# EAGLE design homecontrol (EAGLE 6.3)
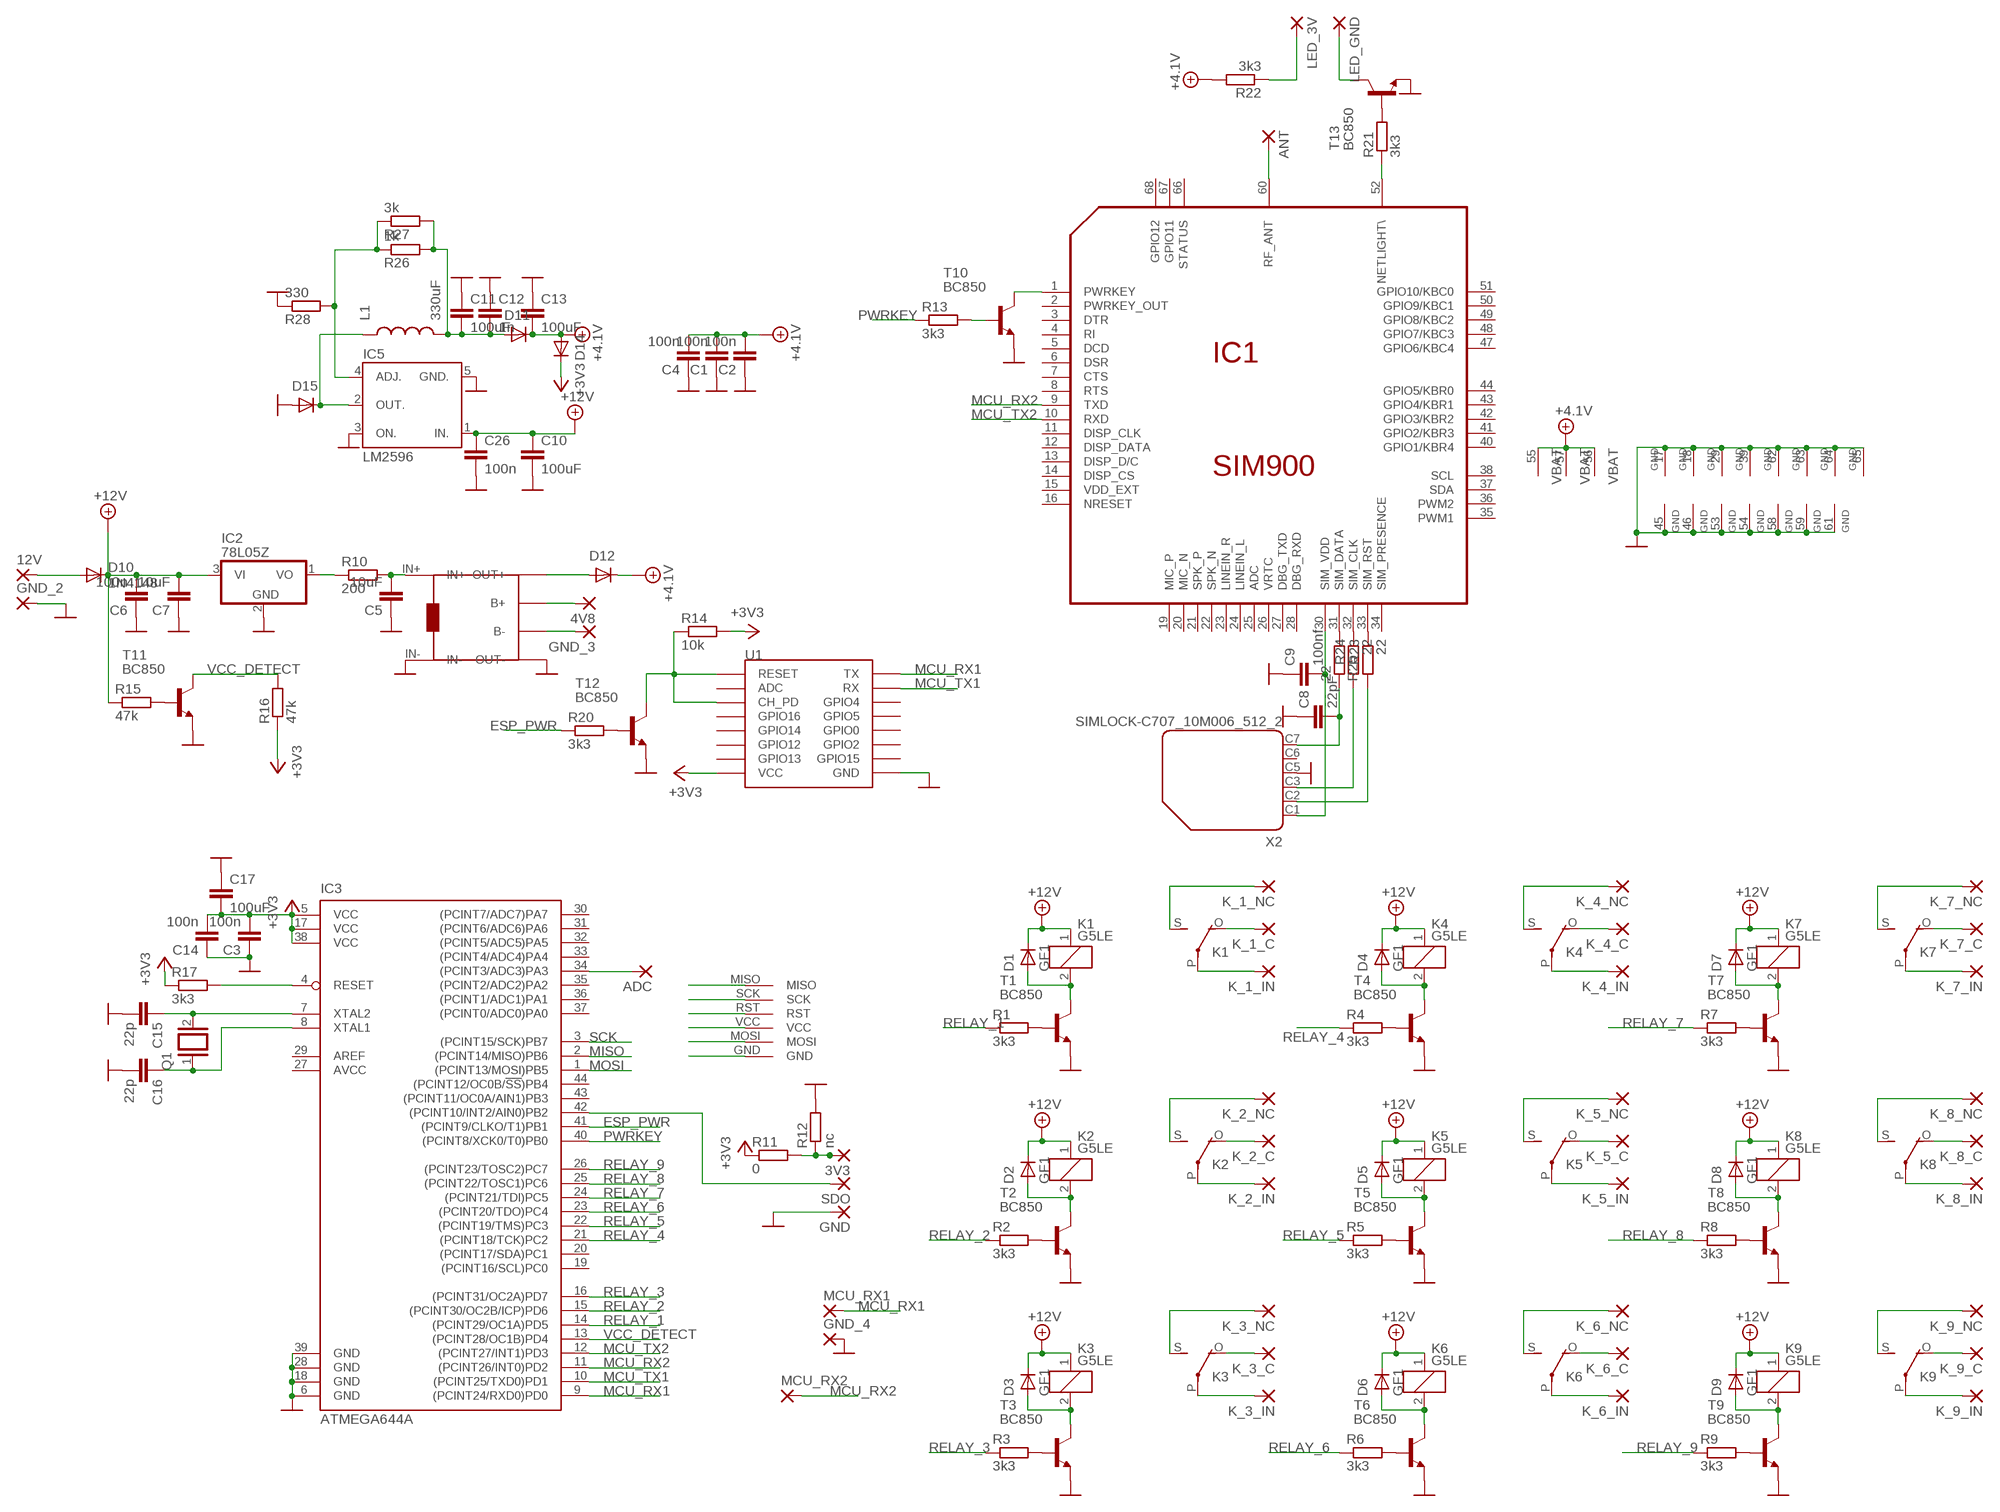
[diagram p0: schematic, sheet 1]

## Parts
3V3  2,15/1,0  [2,15/1,0]
4V8  WIREPAD2,15/1,0  [2,15/1,0]
12V  2,54/0,8  [2,54/0,8]
ADC  SMD2  [SMD1,27-2,54]
ANT  2,54/0,8  [2,54/0,8]
C1  100n  C-EUC1206  [C1206]
C2  100n  C-EUC1206  [C1206]
C3  100n  C-EUC1206  [C1206]
C4  100n  C-EUC1206  [C1206]
C5  10uF  C-EUC1206  [C1206]
C6  100n  C-EUC1206  [C1206]
C7  10uF  C-EUC1206  [C1206]
C8  22pF  C-EUC1206K  [C1206K]
C9  100nf  C-EUC1206K  [C1206K]
C10  100uF  SMD-CAP  [SMD-CAP]
C11  100uF  SMD-CAP  [SMD-CAP]
C12  1n  C-EUC1206K  [C1206K]
C13  100uF  SMD-CAP  [SMD-CAP]
C14  100n  C-EUC1206  [C1206]
C15  22p  C-EUC1206  [C1206]
C16  22p  C-EUC1206  [C1206]
C17  100uF  SMD-CAP  [SMD-CAP]
C26  100n  C-EUC1206K  [C1206K]
D1  GF1  [SMA-DO214AC]
D2  GF1  [SMA-DO214AC]
D3  GF1  [SMA-DO214AC]
D4  GF1  [SMA-DO214AC]
D5  GF1  [SMA-DO214AC]
D6  GF1  [SMA-DO214AC]
D7  GF1  [SMA-DO214AC]
D8  GF1  [SMA-DO214AC]
D9  GF1  [SMA-DO214AC]
D10  1N4148  1N4148DO35-10  [DO35-10]
D11  GF1  [SMA-DO214AC]
D12  GF1  [SMA-DO214AC]
D14  GF1  [SMA-DO214AC]
D15  GF1  [SMA-DO214AC]
GND  2,54/0,8  [2,54/0,8]
GND_2  2,15/1,0  [2,15/1,0]
GND_3  2,15/1,0  [2,15/1,0]
GND_4  2,15/1,0  [2,15/1,0]
IC1  SIM900  [SIM900]
IC2  78L05Z  [TO92]
IC3  ATMEGA644A  [TQFP44]
IC5  LM2596  LM2931S-ADJ  [TO263-5]
K1  G5LE  [G5LE]
K2  G5LE  [G5LE]
K3  G5LE  [G5LE]
K4  G5LE  [G5LE]
K5  G5LE  [G5LE]
K6  G5LE  [G5LE]
K7  G5LE  [G5LE]
K8  G5LE  [G5LE]
K9  G5LE  [G5LE]
K_1_C  2,54/0,8  [2,54/0,8]
K_1_IN  2,54/0,8  [2,54/0,8]
K_1_NC  2,54/0,8  [2,54/0,8]
K_2_C  2,54/0,8  [2,54/0,8]
K_2_IN  2,54/0,8  [2,54/0,8]
K_2_NC  2,54/0,8  [2,54/0,8]
K_3_C  2,54/0,8  [2,54/0,8]
K_3_IN  2,54/0,8  [2,54/0,8]
K_3_NC  2,54/0,8  [2,54/0,8]
K_4_C  2,54/0,8  [2,54/0,8]
K_4_IN  2,54/0,8  [2,54/0,8]
K_4_NC  2,54/0,8  [2,54/0,8]
K_5_C  2,54/0,8  [2,54/0,8]
K_5_IN  2,54/0,8  [2,54/0,8]
K_5_NC  2,54/0,8  [2,54/0,8]
K_6_C  2,54/0,8  [2,54/0,8]
K_6_IN  2,54/0,8  [2,54/0,8]
K_6_NC  2,54/0,8  [2,54/0,8]
K_7_C  2,54/0,8  [2,54/0,8]
K_7_IN  2,54/0,8  [2,54/0,8]
K_7_NC  2,54/0,8  [2,54/0,8]
K_8_C  2,54/0,8  [2,54/0,8]
K_8_IN  2,54/0,8  [2,54/0,8]
K_8_NC  2,54/0,8  [2,54/0,8]
K_9_C  2,54/0,8  [2,54/0,8]
K_9_IN  2,54/0,8  [2,54/0,8]
K_9_NC  2,54/0,8  [2,54/0,8]
L1  330uF  SMD-INDUCTOR  [SMD-COIL]
LED_3V  WIREPAD2,15/1,0  [2,15/1,0]
LED_GND  WIREPAD2,15/1,0  [2,15/1,0]
MCU_RX1  2,15/1,0  [2,15/1,0]
MCU_RX2  2,15/1,0  [2,15/1,0]
Q1  XTAL/S  [QS]
R1  3k3  R-EU_M3216  [M3216]
R2  3k3  R-EU_M3216  [M3216]
R3  3k3  R-EU_M3216  [M3216]
R4  3k3  R-EU_M3216  [M3216]
R5  3k3  R-EU_M3216  [M3216]
R6  3k3  R-EU_M3216  [M3216]
R7  3k3  R-EU_M3216  [M3216]
R8  3k3  R-EU_M3216  [M3216]
R9  3k3  R-EU_M3216  [M3216]
R10  200  R-EU_M3216  [M3216]
R11  0  R-EU_M3216  [M3216]
R12  nc  R-EU_M3216  [M3216]
R13  3k3  R-EU_M3216  [M3216]
R14  10k  R-EU_M3216  [M3216]
R15  47k  R-EU_M3216  [M3216]
R16  47k  R-EU_M3216  [M3216]
R17  3k3  R-EU_M3216  [M3216]
R20  3k3  R-EU_M3216  [M3216]
R21  3k3  R-EU_M3216  [M3216]
R22  3k3  R-EU_M3216  [M3216]
R23  22  R-EU_M1206  [M1206]
R24  22  R-EU_M1206  [M1206]
R25  22  R-EU_M1206  [M1206]
R26  1k  R-EU_M3216  [M3216]
R27  3k  R-EU_M3216  [M3216]
R28  330  R-EU_M3216  [M3216]
SDO  2,15/1,0  [2,15/1,0]
T1  BC850  [SOT23]
T2  BC850  [SOT23]
T3  BC850  [SOT23]
T4  BC850  [SOT23]
T5  BC850  [SOT23]
T6  BC850  [SOT23]
T7  BC850  [SOT23]
T8  BC850  [SOT23]
T9  BC850  [SOT23]
T10  BC850  [SOT23]
T11  BC850  [SOT23]
T12  BC850  [SOT23]
T13  BC850  [SOT23]
U1  ESP12SMD  [ESP12-SMD]
U$1  AVR_ISP  [AVR_ISP]
U$2  AKUTOLTO  [AKUTOLTO]
X2  SIMLOCK-C707_10M006_512_2  [C707_10M006_512_2]

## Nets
+3V3: C3.2 C14.2 C17.P$2 D14.K(C) IC3.5(VCC) IC3.17(VCC) IC3.38(VCC) R11.1 R14.2 R16.1 R17.1 U1.VCC U$1.VCC
+4.1V: C1.2 C2.2 C4.2 C13.P$2 D11.K(C) D12.K(C) D14.A IC1.55(VBAT) IC1.56(VBAT) IC1.57(VBAT) R22.2
+12V: C6.2 C7.2 C10.P$1 C26.1 D1.K(C) D2.K(C) D3.K(C) D4.K(C) D5.K(C) D6.K(C) D7.K(C) D8.K(C) D9.K(C) D10.C IC2.3(VI) IC5.1(IN.) K1.1 K2.1 K3.1 K4.1 K5.1 K6.1 K7.1 K8.1 K9.1 R15.1
ESP_PWR: IC3.41((PCINT9/CLKO/T1)PB1) R20.1
GND: C1.1 C2.1 C3.1 C4.1 C5.1 C6.1 C7.1 C8.1 C9.1 C10.P$2 C11.P$1 C12.1 C13.P$1 C14.1 C15.2 C16.2 C17.P$1 C26.2 D15.A GND.1(P) GND_2.1(P) GND_4.1(P) IC1.17(GND) IC1.18(GND) IC1.29(GND) IC1.39(GND) IC1.45(GND) IC1.46(GND) IC1.53(GND) IC1.54(GND) IC1.58(GND) IC1.59(GND) IC1.61(GND) IC1.62(GND) IC1.63(GND) IC1.64(GND) IC1.65(GND) IC2.2(GND) IC3.6(GND) IC3.18(GND) IC3.28(GND) IC3.39(GND) IC5.3(ON.) IC5.5(GND.) R12.2 R28.1 T1.2(E) T2.2(E) T3.2(E) T4.2(E) T5.2(E) T6.2(E) T7.2(E) T8.2(E) T9.2(E) T10.2(E) T11.2(E) T12.2(E) T13.2(E) U1.GND U$1.GND U$2.IN- U$2.OUT- X2.C5
MCU_RX1: IC3.9((PCINT24/RXD0)PD0) MCU_RX1.1(P) U1.TXD0(TX)
MCU_RX2: IC1.9(TXD) IC3.11((PCINT26/INT0)PD2) MCU_RX2.1(P)
MCU_TX1: IC3.10((PCINT25/TXD0)PD1) U1.RXD0(RX)
MCU_TX2: IC1.10(RXD) IC3.12((PCINT27/INT1)PD3)
MISO: IC3.2((PCINT14/MISO)PB6) U$1.MISO
MOSI: IC3.1((PCINT13/MOSI)PB5) U$1.MOSI
N$1: R1.2 T1.1(B)
N$2: D1.A K1.2 T1.3(C)
N$3: K1.S(2:S) K_1_NC.1(P)
N$4: K1.P(2:P) K_1_IN.1(P)
N$5: K1.O(2:O) K_1_C.1(P)
N$6: R2.2 T2.1(B)
N$7: D2.A K2.2 T2.3(C)
N$8: K2.P(2:P) K_2_IN.1(P)
N$9: K2.O(2:O) K_2_C.1(P)
N$10: K2.S(2:S) K_2_NC.1(P)
N$11: R3.2 T3.1(B)
N$12: D3.A K3.2 T3.3(C)
N$13: K3.P(2:P) K_3_IN.1(P)
N$14: K3.O(2:O) K_3_C.1(P)
N$15: K3.S(2:S) K_3_NC.1(P)
N$16: R4.2 T4.1(B)
N$17: D4.A K4.2 T4.3(C)
N$18: K4.P(2:P) K_4_IN.1(P)
N$19: K4.O(2:O) K_4_C.1(P)
N$20: K4.S(2:S) K_4_NC.1(P)
N$21: R5.2 T5.1(B)
N$22: D5.A K5.2 T5.3(C)
N$23: K5.P(2:P) K_5_IN.1(P)
N$24: K5.O(2:O) K_5_C.1(P)
N$25: K5.S(2:S) K_5_NC.1(P)
N$26: R6.2 T6.1(B)
N$27: D6.A K6.2 T6.3(C)
N$28: K6.P(2:P) K_6_IN.1(P)
N$29: K6.O(2:O) K_6_C.1(P)
N$30: K6.S(2:S) K_6_NC.1(P)
N$31: R7.2 T7.1(B)
N$32: D7.A K7.2 T7.3(C)
N$33: K7.P(2:P) K_7_IN.1(P)
N$34: K7.O(2:O) K_7_C.1(P)
N$35: K7.S(2:S) K_7_NC.1(P)
N$36: R8.2 T8.1(B)
N$37: D8.A K8.2 T8.3(C)
N$38: K8.P(2:P) K_8_IN.1(P)
N$39: K8.O(2:O) K_8_C.1(P)
N$40: K8.S(2:S) K_8_NC.1(P)
N$41: R9.2 T9.1(B)
N$42: D9.A K9.2 T9.3(C)
N$43: K9.P(2:P) K_9_IN.1(P)
N$44: K9.O(2:O) K_9_C.1(P)
N$45: K9.S(2:S) K_9_NC.1(P)
N$46: C5.2 R10.2 U$2.IN+
N$47: D12.A U$2.OUT+
N$48: IC2.1(VO) R10.1
N$49: IC3.42((PCINT10/INT2/AIN0)PB2) SDO.1(P)
N$50: 3V3.1(P) R11.2 R12.1
N$51: R13.2 T10.1(B)
N$52: IC1.1(PWRKEY) T10.3(C)
N$53: D15.K(C) IC5.2(OUT.) L1.P$1
N$54: 12V.1(P) D10.A
N$55: R14.1 T12.3(C) U1.CH_PD U1.RESET
N$56: 4V8.1(P) U$2.B+
N$57: R15.2 T11.1(B)
N$58: GND_3.1(P) U$2.B-
N$60: C11.P$2 C12.2 D11.A L1.P$2 R26.2 R27.2
N$61: C15.1 IC3.7(XTAL2) Q1.2
N$62: R20.2 T12.1(B)
N$63: IC5.4(ADJ.) R26.1 R27.1 R28.2
N$64: ANT.1(P) IC1.60(RF_ANT)
N$65: IC1.52(NETLIGHT\) R21.1
N$66: R21.2 T13.1(B)
N$67: LED_GND.1(P) T13.3(C)
N$68: LED_3V.1(P) R22.1
N$69: C9.2 IC1.30(SIM_VDD) X2.C1
N$70: R23.2 X2.C2
N$71: R24.2 X2.C3
N$72: C8.2 R25.1 X2.C7
N$73: IC1.33(SIM_RST) R23.1
N$74: IC1.32(SIM_CLK) R24.1
N$75: IC1.31(SIM_DATA) R25.2
N$79: C16.1 IC3.8(XTAL1) Q1.1
N$80: ADC.1(P) IC3.34((PCINT3/ADC3)PA3)
PWRKEY: IC3.40((PCINT8/XCK0/T0)PB0) R13.1
RELAY_1: IC3.14((PCINT29/OC1A)PD5) R1.1
RELAY_2: IC3.15((PCINT30/OC2B/ICP)PD6) R2.1
RELAY_3: IC3.16((PCINT31/OC2A)PD7) R3.1
RELAY_4: IC3.21((PCINT18/TCK)PC2) R4.1
RELAY_5: IC3.22((PCINT19/TMS)PC3) R5.1
RELAY_6: IC3.23((PCINT20/TDO)PC4) R6.1
RELAY_7: IC3.24((PCINT21/TDI)PC5) R7.1
RELAY_8: IC3.25((PCINT22/TOSC1)PC6) R8.1
RELAY_9: IC3.26((PCINT23/TOSC2)PC7) R9.1
RESET: IC3.4(RESET) R17.2 U$1.RST
SCK: IC3.3((PCINT15/SCK)PB7) U$1.SCK
VCC_DETECT: IC3.13((PCINT28/OC1B)PD4) R16.2 T11.3(C)
Unconnected: IC1.2(PWRKEY_OUT) IC1.3(DTR) IC1.4(RI) IC1.5(DCD) IC1.6(DSR) IC1.7(CTS) IC1.8(RTS) IC1.11(DISP_CLK) IC1.12(DISP_DATA) IC1.13(DISP_D/C) IC1.14(DISP_CS) IC1.15(VDD_EXT) IC1.16(NRESET) IC1.19(MIC_P) IC1.20(MIC_N) IC1.21(SPK_P) IC1.22(SPK_N) IC1.23(LINEIN_R) IC1.24(LINEIN_L) IC1.25(ADC) IC1.26(VRTC) IC1.27(DBG_TXD) IC1.28(DBG_RXD) IC1.34(SIM_PRESENCE) IC1.35(PWM1) IC1.36(PWM2) IC1.37(SDA) IC1.38(SCL) IC1.40(GPIO1/KBR4) IC1.41(GPIO2/KBR3) IC1.42(GPIO3/KBR2) IC1.43(GPIO4/KBR1) IC1.44(GPIO5/KBR0) IC1.47(GPIO6/KBC4) IC1.48(GPIO7/KBC3) IC1.49(GPIO8/KBC2) IC1.50(GPIO9/KBC1) IC1.51(GPIO10/KBC0) IC1.66(STATUS) IC1.67(GPIO11) IC1.68(GPIO12) IC3.19((PCINT16/SCL)PC0) IC3.20((PCINT17/SDA)PC1) IC3.29(AREF) IC3.30((PCINT7/ADC7)PA7) IC3.31((PCINT6/ADC6)PA6) IC3.32((PCINT5/ADC5)PA5) IC3.33((PCINT4/ADC4)PA4) IC3.35((PCINT2/ADC2)PA2) IC3.36((PCINT1/ADC1)PA1) IC3.37((PCINT0/ADC0)PA0) IC3.43((PCINT11/OC0A/AIN1)PB3) IC3.44((PCINT12/OC0B/!SS!)PB4) U1.ADC U1.GPIO0 U1.GPIO2 U1.GPIO4 U1.GPIO5 U1.GPIO12 U1.GPIO13 U1.GPIO14 U1.GPIO15 U1.GPIO16 X2.C6

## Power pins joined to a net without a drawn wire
AVCC: IC3.27(AVCC)

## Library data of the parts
3V3 GND_2-GND_4 MCU_RX1 MCU_RX2 SDO = wirepad:2,15/1,0: THROUGH-HOLE PAD
4V8 LED_3V LED_GND = wirepad:WIREPAD: Wire PAD connect wire on PCB
12V ANT GND K_1_C K_1_IN K_1_NC K_2_C K_2_IN K_2_NC K_3_C K_3_IN K_3_NC K_4_C K_4_IN K_4_NC K_5_C K_5_IN K_5_NC K_6_C K_6_IN K_6_NC K_7_C K_7_IN K_7_NC K_8_C K_8_IN K_8_NC K_9_C K_9_IN K_9_NC = wirepad:2,54/0,8: THROUGH-HOLE PAD
ADC = wirepad:SMD2: SMD PAD
C1-C7 C14-C16 = resistor:C-EU: CAPACITOR, European symbol
C8 C9 C12 C26 = rcl:C-EU: CAPACITOR, European symbol
C10 C11 C13 C17 = Tomi's_Library:SMD-CAP
D1-D9 D11 D12 D14 D15 = diode:GF1: DIODE
D10 = diode:1N4148: DIODE
IC1 = sim900:SIM900
IC2 = linear:78*: Positive VOLTAGE REGULATOR Source: http://cache.national.com/ds/LM/LM78L05.pdf http://www.fairchildsemi.com/ds/LM/LM7805.pdf
IC3 = atmel:ATMEGA644: 8-bit Microcontroller with 64K Bytes In-System Programmable Flash Source: http://www.atmel.com/dyn/resources/prod_documents/doc2593.pdf; MPN: ATMEGA644PV-10AU; OC_FARNELL: 1455123; OC_NEWARK: 58M3748
IC5 = regulator:LM2931?-ADJ: National Semiconductor Low Dropout Adjustable Regulator Vout 3-24V, Vin up to 26V, Shutdown Pin, Reverse Batterie/Load Dump/Short Circuit/Overload Protection,
K1-K9 = relay:G5LE: RELAY 1 x switch, 10 A/120 V AC, 8 A/30 V DC, Omron; OC_FARNELL: unknown; OC_NEWARK: unknown
L1 = Tomi's_Library:SMD-INDUCTOR
Q1 = special:XTAL/S: CRYSTAL
R1-R17 R20-R22 = rcl:R-EU_: RESISTOR, European symbol
R23-R28 = resistor:R-EU_: RESISTOR, European symbol
T1-T13 = transistor:BC850: NPN TRANSISTOR
U1 = esp8266modules:ESP12: ESP8266 Wifi module 12
U$1 = 2 - csatlakozo:AVR_ISP
U$2 = aksitolto:AKUTOLTO
X2 = con-amphenol:SIMLOCK-C707_10M006_512_2: C707A SIMLOCK® 2.5 mm with wide solder tails Source: Data sheet; OC_FARNELL: unknown; OC_NEWARK: unknown

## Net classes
0 default: clearance 0.355 mm

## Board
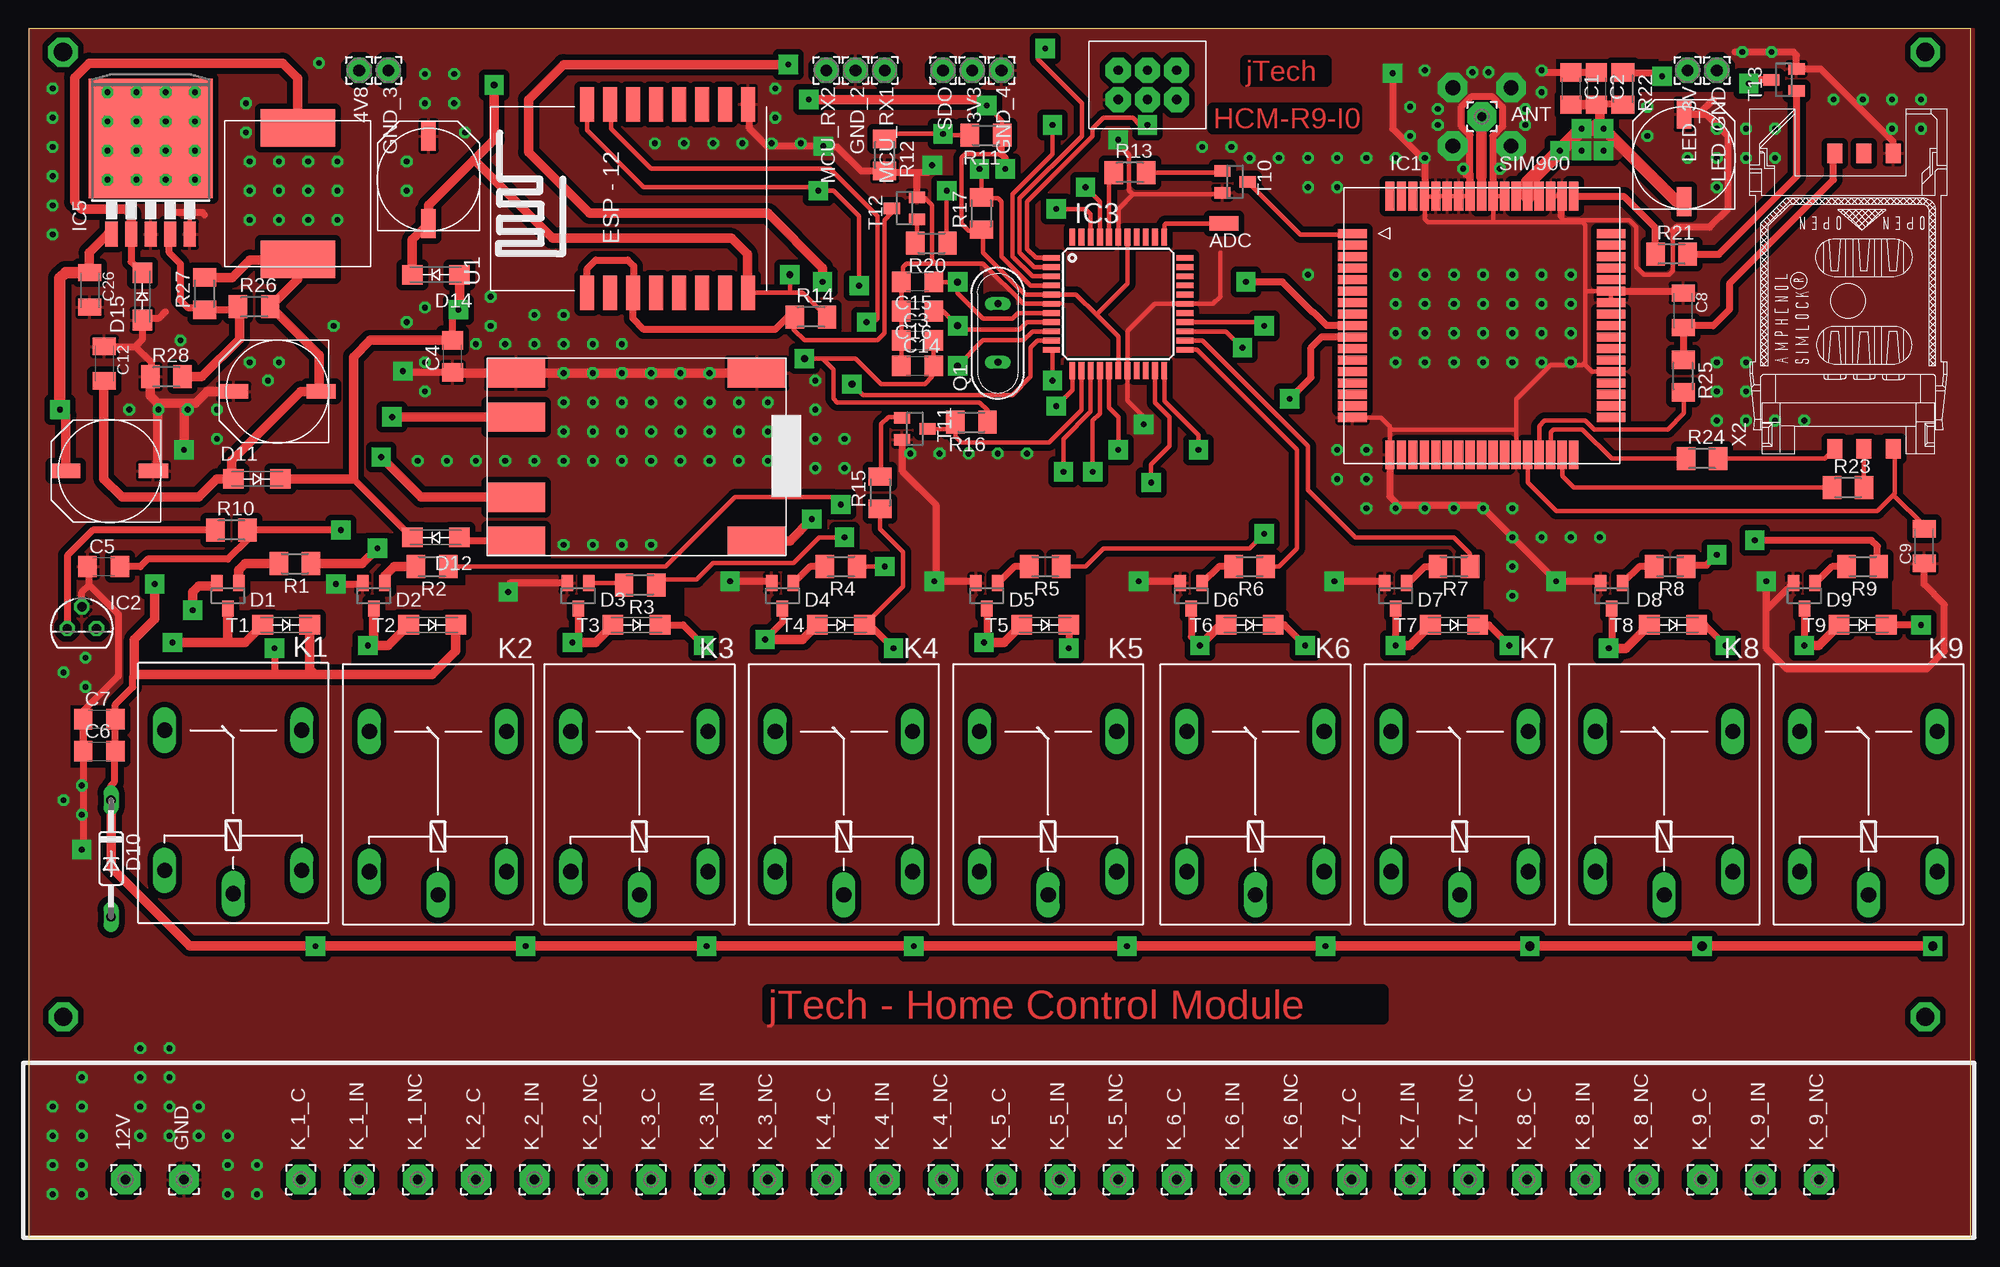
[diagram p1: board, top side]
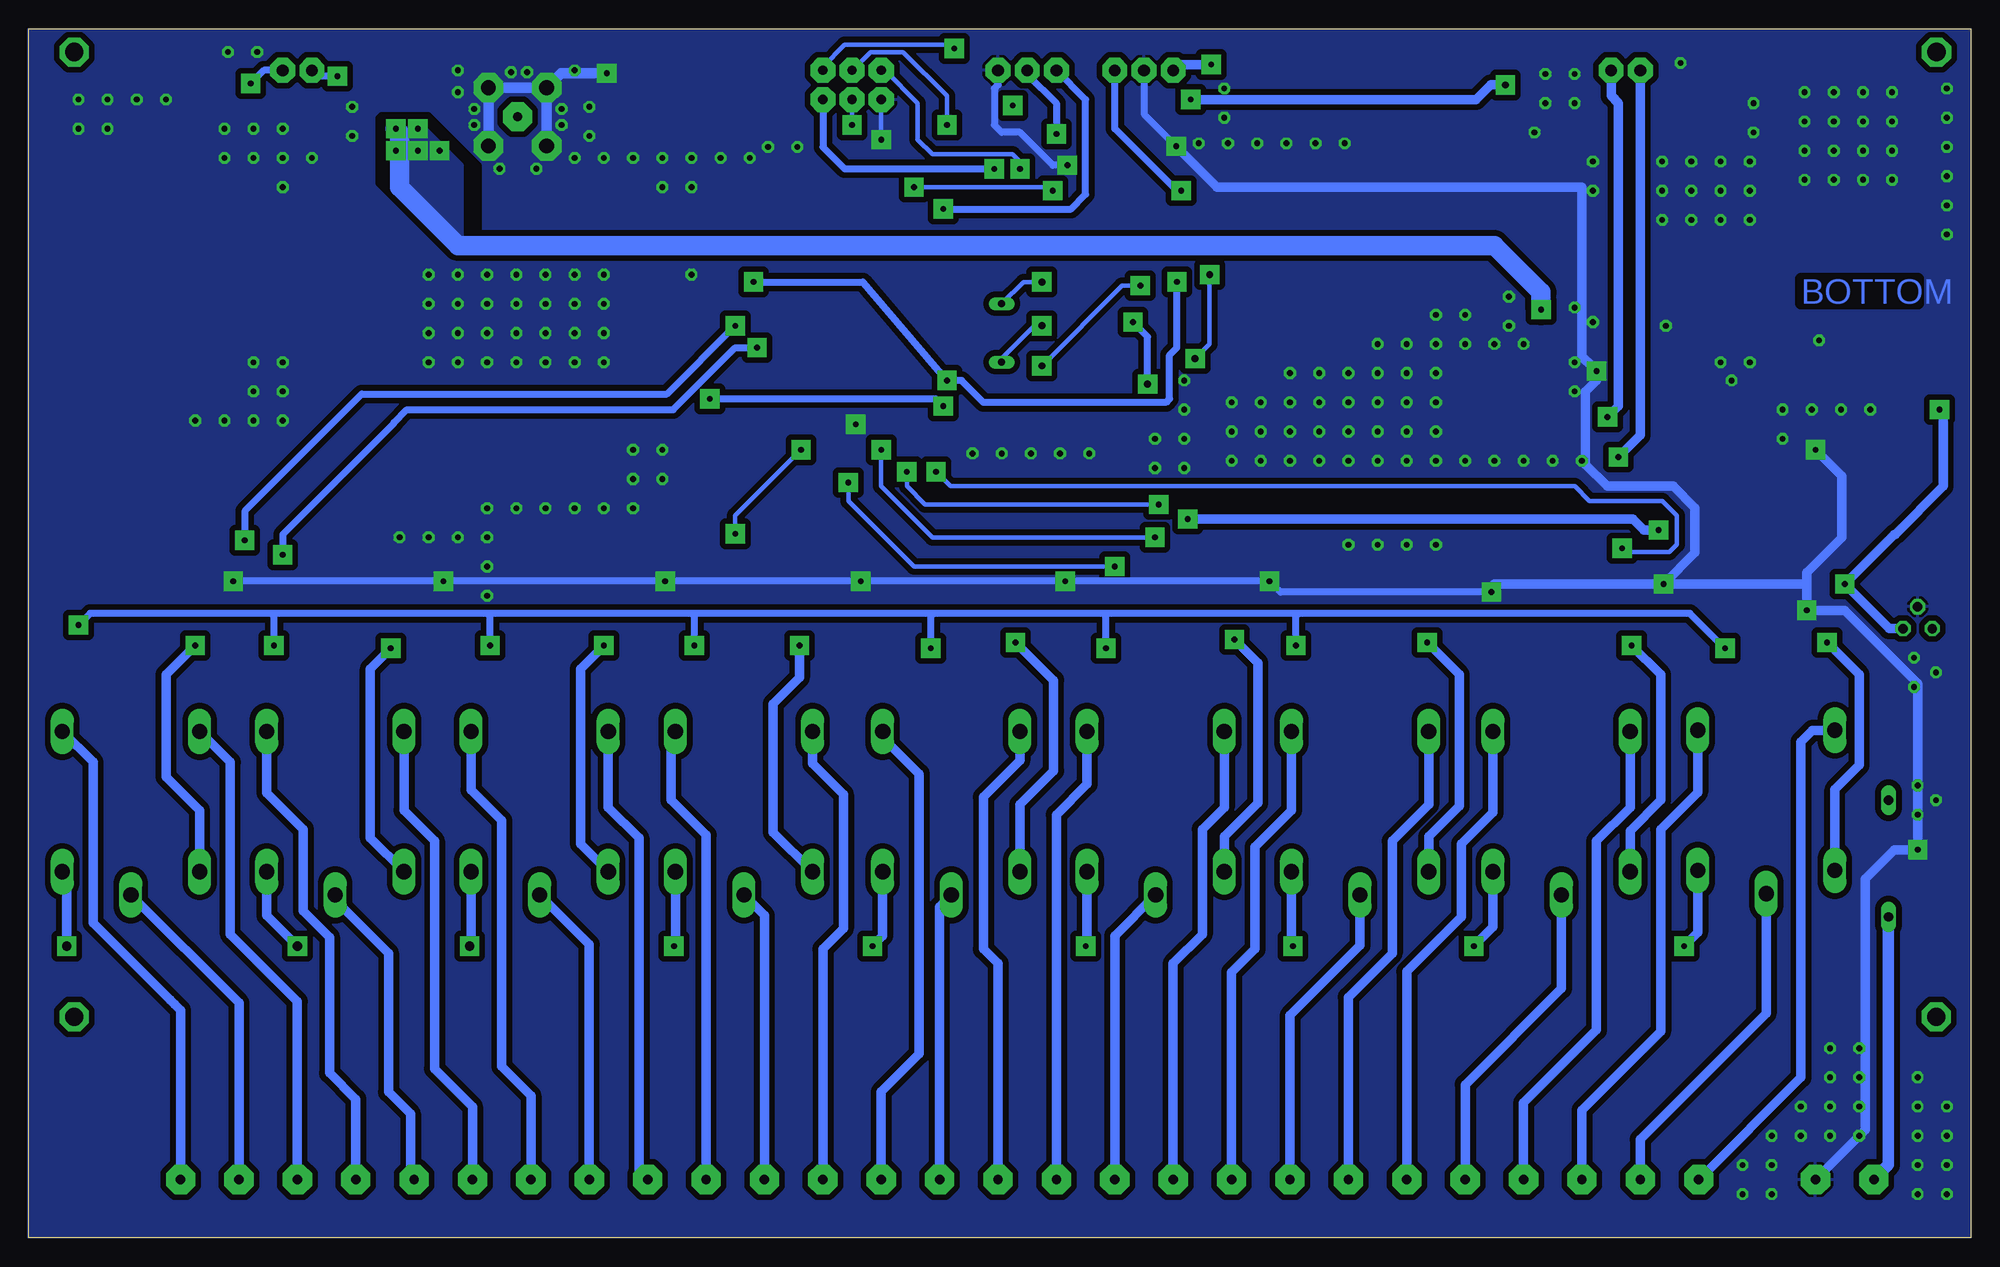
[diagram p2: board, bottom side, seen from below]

Size 168.96 x 105.22 mm. Coordinates in mm from the lower left corner, seen from the top.
Outline: 0,0 168.96,0 168.96,105.22 0,105.22 0,0
Copper layers (1*16): Top 0.035mm / dielectric 1.5mm / Bottom 0.035mm
Design rules "default *": minimum track width 10mil, minimum drill 24mil, track to track 20mil, track to pad 20mil, pad to pad 20mil, via to via 20mil, smd to smd 20mil, copper to edge 0mil, drill to drill 8mil, minimum pad ring 10mil, minimum via ring 8mil, stop-mask expansion 4mil, vias tented up to drill 0mil, thermal gap 10mil
tRestrict: area 11.3,52.7 to 17.3,58.7; area 4,41 to 7.5,46; area 4,41 to 7.5,46.4; area 3.7,41 to 4.9,46.4; area 133.2,99.4 to 138.3,102.6; area 135.4,101.6 to 141.8,102.6; area 132.9,95.6 to 133.5,102.6; area 137.5,99.7 to 149.8,101.2; area 74.8,75.6 to 83,84.1; area 73.2,75.6 to 83,77.2; area 75.1,83.8 to 82.7,89.9; area 18.6,59.1 to 28.1,61.3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
bRestrict: 6 lines

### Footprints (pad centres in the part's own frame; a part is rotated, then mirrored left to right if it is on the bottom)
2,15/1,0 = drill 1.016 pad 2.159 octagon: 1 0,0
2,54/0,8 = drill 0.813 pad 2.54 octagon: 1 0,0
SMD1,27-2,54 = smd 1.27 x 2.54: 1 0,0
C1206 = smd 1.6 x 1.8: 1 -1.4,0; 2 1.4,0
C1206K = smd 1.5 x 2: 1 -1.5,0; 2 1.5,0
SMD-CAP = smd 1.27 x 2.54: P$1 0,3.81; P$2 0,-3.81
SMA-DO214AC = smd 1.8 x 1.7: A -2.05,0; K 2.05,0
DO35-10 = drill 0.813 long: A 5.08,0; C -5.08,0
SIM900 = smd 2.5 x 0.8: 1 -11.25,8; 2 -11.25,7; 3 -11.25,6; 4 -11.25,5; 5 -11.25,4; 6 -11.25,3; 7 -11.25,2; 8 -11.25,1; 9 -11.25,0; 10 -11.25,-1; 11 -11.25,-2; 12 -11.25,-3; 13 -11.25,-4; 14 -11.25,-5; 15 -11.25,-6; 16 -11.25,-7; 17 -11.25,-8; 35 11.25,-8; 36 11.25,-7; 37 11.25,-6; 38 11.25,-5; 39 11.25,-4; 40 11.25,-3; 41 11.25,-2; 42 11.25,-1; 43 11.25,0; 44 11.25,1; 45 11.25,2; 46 11.25,3; 47 11.25,4; 48 11.25,5; 49 11.25,6; 50 11.25,7; 51 11.25,8 | smd 0.8 x 2.5: 18 -8,-11.25; 19 -7,-11.25; 20 -6,-11.25; 21 -5,-11.25; 22 -4,-11.25; 23 -3,-11.25; 24 -2,-11.25; 25 -1,-11.25; 26 0,-11.25; 27 1,-11.25; 28 2,-11.25; 29 3,-11.25; 30 4,-11.25; 31 5,-11.25; 32 6,-11.25; 33 7,-11.25; 34 8,-11.25; 52 8,11.25; 53 7,11.25; 54 6,11.25; 55 5,11.25; 56 4,11.25; 57 3,11.25; 58 2,11.25; 59 1,11.25; 60 0,11.25; 61 -1,11.25; 62 -2,11.25; 63 -3,11.25; 64 -4,11.25; 65 -5,11.25; 66 -6,11.25; 67 -7,11.25; 68 -8,11.25
TO92 = drill 0.813 octagon: 1 -1.27,0; 2 0,1.905; 3 1.27,0
TQFP44 = smd 1.5 x 0.5: 1 -5.8,4; 2 -5.8,3.2; 3 -5.8,2.4; 4 -5.8,1.6; 5 -5.8,0.8; 6 -5.8,0; 7 -5.8,-0.8; 8 -5.8,-1.6; 9 -5.8,-2.4; 10 -5.8,-3.2; 11 -5.8,-4; 23 5.8,-4; 24 5.8,-3.2; 25 5.8,-2.4; 26 5.8,-1.6; 27 5.8,-0.8; 28 5.8,0; 29 5.8,0.8; 30 5.8,1.6; 31 5.8,2.4; 32 5.8,3.2; 33 5.8,4 | smd 0.5 x 1.5: 12 -4,-5.8; 13 -3.2,-5.8; 14 -2.4,-5.8; 15 -1.6,-5.8; 16 -0.8,-5.8; 17 0,-5.8; 18 0.8,-5.8; 19 1.6,-5.8; 20 2.4,-5.8; 21 3.2,-5.8; 22 4,-5.8; 34 4,5.8; 35 3.2,5.8; 36 2.4,5.8; 37 1.6,5.8; 38 0.8,5.8; 39 0,5.8; 40 -0.8,5.8; 41 -1.6,5.8; 42 -2.4,5.8; 43 -3.2,5.8; 44 -4,5.8
TO263-5 = smd 1.067 x 2.159: 1 -3.404,-5.791; 2 -1.702,-5.791; 3 0,-5.791; 4 1.702,-5.791; 5 3.404,-5.791 | smd 10.8 x 10.41: 6 0,2.54
G5LE = drill 1.321 long: 1 -7.493,-5.969; 2 -7.493,5.969; O 4.699,5.969; P -9.525,0; S 4.699,-5.969
SMD-COIL = smd 6.452 x 3.251: P$1 0,5.715; P$2 0,-5.715
QS = drill 0.61 long: 1 -2.54,0; 2 2.54,0
M3216 = smd 1.6 x 2: 1 -1.4,0; 2 1.4,0
M1206 = smd 1.6 x 2: 1 -1.4,0; 2 1.4,0
SOT23 = smd 1 x 1.4: 1 -0.95,-1.1; 2 0.95,-1.1; 3 0,1.1
ESP12-SMD = smd 3 x 1.2: ADC -8.3,3.8; CH_PD -8.3,1.8; GND 8.1,-8.2; GPIO0 8.1,-2.2; GPIO2 8.1,-4.2; GPIO4 8.1,1.8; GPIO5 8.1,-0.2; GPIO12 -8.3,-4.2; GPIO13 -8.3,-6.2; GPIO14 -8.3,-2.2; GPIO15 8.1,-6.2; GPIO16 -8.3,-0.2; RESET -8.3,5.8; RXD0 8.1,3.8; TXD0 8.1,5.8; VCC -8.3,-8.2
AVR_ISP = drill 0.8 pad 2.184 octagon: GND 0,-2.54; MISO -2.54,2.54; MOSI 0,0; RST -2.54,-2.54; SCK -2.54,0; VCC 0,2.54
AKUTOLTO = smd 2.54 x 5.08: B+ -3.81,10.795; B- 3.175,10.795; IN+ -7.62,-10.16; IN- 6.985,-10.16; OUT+ -7.62,10.795; OUT- 6.985,10.795
C707_10M006_512_2 = smd 1.7 x 1.3: C1 -12.85,-3.915; C2 -12.85,-1.375; C3 -12.85,1.165; C5 12.85,-3.915; C6 12.85,-1.375; C7 12.85,1.165

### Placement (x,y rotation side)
3V3  82.09,101.6 180 top
4V8  28.75,101.6 180 top
12V  8.43,5.08 90 top
ADC  104,88.27 90 top
ANT  126.43,97.56 0 top
C1  134.16,100.01 270 top
C2  136.38,100.01 270 top
C3  77.33,78.11 0 top
C4  36.88,76.71 90 top
C5  6.53,58.42 0 top
C6  6.14,42.35 0 top
C7  6.14,45.15 0 top
C8  143.94,80.71 270 top
C9  164.89,60.2 90 top
C10  7.03,66.74 90 top
C11  21.64,73.66 90 top
C12  6.59,76.07 270 top
C13  144,93.98 0 top
C14  77.33,75.88 0 top
C15  77.33,83.18 180 top
C16  77.33,80.64 180 top
C17  34.78,92.07 0 top
C26  5.32,82.49 270 top
D1  22.4,53.34 0 top
D2  35.1,53.34 0 top
D3  52.88,53.34 0 top
D4  70.66,53.34 0 top
D5  88.44,53.34 0 top
D6  106.22,53.34 0 top
D7  124,53.34 0 top
D8  143.05,53.34 0 top
D9  159.56,53.34 0 top
D10  7.16,33.02 270 top
D11  19.86,66.04 0 top
D12  35.42,60.96 180 top
D14  35.42,83.82 180 top
D15  9.89,81.91 90 top
GND  13.51,5.08 90 top
GND_2  71.93,101.6 180 top
GND_3  31.29,101.6 180 top
GND_4  84.63,101.6 180 top
IC1  126.41,79.4 0 top
IC2  4.62,53.02 0 top
IC3  94.79,81.28 0 top
IC5  10.61,93.12 0 top
K1  17.79,39.48 90 top
K2  35.61,39.37 90 top
K3  53.13,39.37 90 top
K4  70.91,39.37 90 top
K5  88.69,39.37 90 top
K6  106.73,39.37 90 top
K7  124.51,39.37 90 top
K8  142.29,39.37 90 top
K9  160.07,39.37 90 top
K_1_C  23.67,5.08 90 top
K_1_IN  28.75,5.08 90 top
K_1_NC  33.83,5.08 90 top
K_2_C  38.91,5.08 90 top
K_2_IN  43.99,5.08 90 top
K_2_NC  49.07,5.08 90 top
K_3_C  54.15,5.08 90 top
K_3_IN  59.23,5.08 90 top
K_3_NC  64.31,5.08 90 top
K_4_C  69.39,5.08 90 top
K_4_IN  74.47,5.08 90 top
K_4_NC  79.55,5.08 90 top
K_5_C  84.63,5.08 90 top
K_5_IN  89.71,5.08 90 top
K_5_NC  94.79,5.08 90 top
K_6_C  99.87,5.08 90 top
K_6_IN  104.95,5.08 90 top
K_6_NC  110.03,5.08 90 top
K_7_C  115.11,5.08 90 top
K_7_IN  120.19,5.08 90 top
K_7_NC  125.27,5.08 90 top
K_8_C  130.35,5.08 90 top
K_8_IN  135.43,5.08 90 top
K_8_NC  140.51,5.08 90 top
K_9_C  145.59,5.08 90 top
K_9_IN  150.67,5.08 90 top
K_9_NC  155.75,5.08 90 top
L1  23.42,90.87 0 top
LED_3V  144.32,101.6 180 top
LED_GND  146.86,101.6 180 top
MCU_RX1  74.47,101.6 180 top
MCU_RX2  69.39,101.6 180 top
Q1  84.31,78.74 90 top
R1  23.16,58.67 180 top
R2  35.1,58.42 180 top
R3  53.2,56.83 180 top
R4  70.66,58.42 180 top
R5  88.44,58.42 180 top
R6  106.22,58.42 180 top
R7  124,58.42 180 top
R8  142.8,58.42 180 top
R9  159.56,58.42 180 top
R10  17.64,61.59 0 top
R11  83.28,95.94 180 top
R12  74.47,94.23 270 top
R13  95.81,92.71 0 top
R14  68.06,80.14 0 top
R15  74.08,64.85 90 top
R16  82.01,70.98 180 top
R17  82.88,89.14 90 top
R20  78.53,86.55 180 top
R21  142.92,85.6 0 top
R22  138.7,100.01 270 top
R23  158.29,65.28 0 top
R24  145.59,67.82 0 top
R25  143.94,74.99 270 top
R26  19.61,81.03 0 top
R27  15.29,82.17 90 top
R28  11.99,74.93 0 top
SDO  79.55,101.6 180 top
T1  17.32,55.88 180 top
T2  30.02,55.88 180 top
T3  47.8,55.88 180 top
T4  65.58,55.88 180 top
T5  83.36,55.88 180 top
T6  101.14,55.88 180 top
T7  118.92,55.88 180 top
T8  137.72,55.88 180 top
T9  154.48,55.88 180 top
T10  104.95,91.9 270 top
T11  77.09,70.41 270 top
T12  76.18,89.6 90 top
T13  152.7,100.77 90 top
U1  54.38,90.55 90 top
U$1  97.33,99.06 270 top
U$2  53.2,68.26 90 top
X2  158.29,81.53 90 top

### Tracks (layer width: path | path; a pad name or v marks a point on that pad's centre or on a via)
+3V3  (via drill 0.5 pad 1.68, 0.6 pad 1.68)
  Top 0.406: U1.VCC 66.22,82.25 | 66.22,82.25 67.34,82.25 R14.2 69.58,80.01 | R11.1 84.68,97.23 v83.36,98.55 | IC3.17 94.79,78.42 92.89,80.33 | 92.89,80.33 91.13,82.08 IC3.5 86.69,82.08 83.04,85.72 83.04,87.57 R17.1 82.77,87.63 81.77,87.63 81.14,88.27 81.14,93.98 81.45,94.3 84.63,94.3 | IC3.38 95.59,83.03 92.89,80.33 | C14.2 C3.2 | R16.1 83.41,72.02 82.72,72.71 70.34,72.71 70.03,73.02 70.03,75.56 69.07,76.52 | 79.23,75.75 C14.2 | v66.22,83.82 66.22,82.25 | C14.2 78.6,75.75 78.6,74.93 77.96,74.3 74.15,74.3 71.93,76.52 69.07,76.52 | 69.07,76.52 v67.48,76.52
  Top 0.61: v84.95,93.03 84.95,93.98 84.63,94.3 84.63,95.88 R11.1
  Top 0.813: U1.VCC 62.53,82.3 62.53,85.6 61.14,86.99 45.58,86.99 38.75,93.82 | v83.36,98.55 82.85,99.06 v67.87,99.06 | 38.75,93.82 34.78,89.85 C17.P$2 33.37,86.85 D14.K | 38.75,93.82 40.5,95.57 v40.5,100.33
  Bottom 0.406: v67.48,76.52 66.22,77.79 v66.22,83.82
  Bottom 0.61: U$1.VCC 99.87,94.93 97.97,93.03 v84.95,93.03
  Bottom 0.813: v40.5,100.33 41.77,100.33 43.04,99.06 v67.87,99.06
+4.1V  (via drill 0.5 pad 1.68)
  Top 0.61: IC1.55 IC1.56 IC1.57 | C4.2 36.88,80.26 v37.39,80.77 | 136.32,96.9 136.7,96.52 | 28.26,66.04 28.29,66.04 D12.K | 136.7,98.3 136.7,98.47 136.93,98.7 138.62,98.7 R22.2
  Top 0.813: D11.K 28.26,66.04 28.26,76.66 29.7,78.11 C4.2 | 37.32,80.84 v37.39,80.77 37.47,80.85 D14.A | C1.2 C2.2 136.7,98.3 136.7,96.84 136.64,96.9 136.32,96.9
  Top 1.016: C13.P$2 143.37,90.17 v137.02,96.52
  Top 1.27: IC1.56 130.41,91.82 v133.21,94.61 v135.11,96.52 136.7,96.52 v137.02,96.52 137.08,96.52
  Bottom 1.676: v37.39,80.77 37.39,82.3 41.45,86.36 131.62,86.36 136.7,91.44 136.7,96.14 137.08,96.52
  other vias: 135.11,94.61 137.02,94.61
  pour Bottom: 137.02,96.52 134.48,96.52 131.3,93.34 131.3,86.36 131.62,86.36 136.7,91.44 137.02,91.76
  pour Top: 132.57,93.98 138.29,93.98 138.92,94.61 137.02,96.52 135.11,96.52
+12V  (via drill 0.5 pad 1.68, 0.8 pad 1.68)
  Top 0.406: R15.1 74.08,61.67 76.06,59.69 76.06,56.69 D4.K
  Top 0.61: D5.K 90.49,51.33 v90.47,51.31 | v21.38,51.31 21.38,49.28 21.13,49.02 | D3.K 56.94,53.34 v58.72,51.56 | D4.K 73.2,53.34 v75.23,51.31 | v164.64,53.34 D9.K | D6.K 109.27,53.34 v111.05,51.56 | D7.K 127.05,53.34 v128.83,51.56 | D8.K 145.84,53.34 v147.62,51.56 | 3.03,66.93 C10.P$1 | D10.C 7.16,39.37 7.48,39.69 7.48,42.29 C6.2 C7.2 7.54,46.42 9.06,47.94 9.06,48.9 9.19,49.02
  Top 0.813: D10.C 7.16,32.26 14.02,25.4 v24.94,25.4 v43.23,25.4 v58.98,25.4 v77.01,25.4 v95.55,25.4 v112.82,25.4 v130.6,25.4 v145.59,25.4 v165.66,25.4 | 24.45,52.31 D1.K 24.45,49.51 24.94,49.02 | 24.94,49.02 21.13,49.02 9.19,49.02 9.19,52.07 10.97,53.85 v10.97,56.9 | 24.94,49.02 35.1,49.02 37.13,51.05 37.13,53.32 D2.K | C10.P$1 3.22,71.56 v2.71,72.07 | IC5.1 6.86,87.33 5.26,85.72 5.26,84.05 C26.1
  Top 1.016: C26.1 3.2,83.99 2.71,83.5 v2.71,72.07
  Bottom 0.61: v21.38,51.31 24.43,54.36 58.47,54.36 | v111.05,51.56 111.05,54.1 111.3,54.36 | v128.83,51.56 128.83,54.1 129.08,54.36 | v147.62,51.56 147.62,54.1 147.88,54.36 | 58.47,54.36 75.23,54.36 | 75.23,54.36 90.22,54.36 | 90.22,54.36 111.3,54.36 | 111.3,54.36 129.08,54.36 | 129.08,54.36 147.88,54.36 | 147.88,54.36 163.62,54.36 v164.64,53.34 | v90.47,51.31 90.47,54.1 90.22,54.36 | v58.72,51.56 58.72,54.1 58.47,54.36 | v75.23,51.31 75.23,54.36
  Bottom 0.813: v165.66,25.4 165.66,31.5 K9.1 | K8.1 148.26,28.07 v145.59,25.4 | K7.1 130.48,25.53 v130.6,25.4 | K6.1 112.7,25.53 v112.82,25.4 | K5.1 94.66,26.29 v95.55,25.4 | K4.1 76.88,25.53 v77.01,25.4 | K3.1 59.1,25.53 v58.98,25.4 | K2.1 41.58,27.05 v43.23,25.4 | K1.1 23.76,26.58 v24.94,25.4 | IC2.3 7.1,53.02 v10.97,56.9 6.65,61.21 6.59,61.21 2.4,65.41 2.4,71.75 v2.71,72.07
ESP_PWR  (via drill 0.5 pad 1.68)
  Top 0.406: IC3.41 93.19,90.18 v91.93,91.44 | 79.87,87.63 79.87,86.3 R20.1 79.87,86.93 v79.87,91.12
  Bottom 0.406: v91.93,91.44 79.87,91.44 v79.87,91.12
GND  (via drill 0.5 pad 1.02, 0.5 pad 1.68, 1.3 pad 2.54)
  Top 0.206: 125.43,91.43 125.41,91.41 IC1.61
  Top 0.406: IC1.39 135.98,75.4 135.43,75.95 135.43,76.2 | 135.43,76.2 135.43,82.3 | 135.43,82.3 135.43,88.14 135.18,88.39 133.4,88.39 | 133.4,88.39 127.56,88.39 | 127.56,88.39 121.71,88.39 121.46,88.65 121.46,90.6 | 121.46,90.6 IC1.65 | 121.46,90.6 122.36,90.6 IC1.64 IC1.63 IC1.62 IC1.61 | IC1.58 IC1.59 127.41,88.54 127.56,88.39 | IC1.54 IC1.53 133.41,88.41 133.4,88.39 | IC1.45 IC1.46 135.53,82.4 135.43,82.3 | 135.43,76.2 135.18,75.95 132.38,75.95 129.41,72.98 IC1.29 129.41,70.28 129.33,70.36 118.41,70.36 | IC1.18 118.41,70.36 | 118.41,70.36 118.41,70.61 117.65,71.37 115.19,71.37 IC1.17 | 133.21,90.85 133.21,88.9 133.53,88.58 139.24,88.58 139.88,87.95 139.88,84.45 140.51,83.82 142.73,83.82 143.05,84.14 143.05,87.63 | 96.06,90.8 94.79,89.53 IC3.39 | 96.06,90.8 103.7,90.8 T10.2 | 96.06,90.8 95.74,91.12 95.74,94.3 94.79,95.25 v94.79,95.57 | v97.01,70.8 97.01,71.44 95.59,72.86 IC3.18 95.59,78.91 97.97,81.28 IC3.28 103.05,81.28 103.68,81.91 103.68,85.72 | 89.71,81.28 IC3.6 86.53,81.28 83.04,84.77 78.92,84.77 | C3.1 76.56,78.61 | C3.1 C14.1 | 78.92,84.77 78.6,85.09 78.6,89.85 77.96,90.49 77.35,90.49 T12.2 | C3.1 C16.2 C15.2 76.06,83.31 76.06,84.45 76.38,84.77 78.92,84.77 | IC5.5 14.01,89.08 14.14,89.22
  Top 0.61: T1.2 16.37,56.71 | T9.2 151.18,54.63 v151.18,57.15 151.18,51.31 152.96,49.53 165.15,49.53 166.67,51.05 166.67,55.12 164.89,56.9 C9.1 | 29.07,56.71 T2.2 28.99,56.9 v26.72,56.9 | T3.2 41.87,56.98 41.87,56.37 v41.7,56.2 | IC1.18 118.41,64.52 119.17,63.75 126.29,63.75 v132.89,57.15 136.6,57.15 T8.2 | v118.67,101.35 118.67,96.52 121.46,93.73 121.46,90.7 IC1.65 | v113.59,57.15 117.8,57.15 T7.2 | v96.57,57.15 100.02,57.15 T6.2 | T5.2 82.24,57.15 v78.79,57.15 78.92,57.28 78.92,63.82 75.99,66.74 T11.2 | v61.01,57.15 64.46,57.15 T4.2 | X2.C5 162.21,95.4 155.88,101.72 T13.2 153.8,102.91 153.53,103.19 148.45,103.19 | C4.1 32.69,75.31 v32.56,75.44 | IC1.46 143.75,82.4 C8.1 | 146.54,99.06 145.27,97.79 C13.P$1 145.91,97.79 147.81,95.88 147.81,89.53 146.22,87.95 143.37,87.95 143.05,87.63 | 133.21,90.85 IC1.53 | C12.1 9.28,77.57 | 9.28,77.57 10.65,76.2 10.65,75 R28.1 | 9.28,77.57 9.89,78.18 D15.A 10.04,80.01 11.29,80.01 11.88,80.6 | 15.28,89.03 15.1,89.22 14.14,89.22 12.24,89.22 | IC2.2 4.62,56.2 5.26,56.83 | 5.26,56.83 5.26,58.29 C5.1 | 5.26,56.83 7.79,54.29 7.79,48.9 4.62,45.72 4.62,45.27 C7.1 | C6.1 C7.1 | C7.1 4.74,33.91 v4.62,33.78 | v78.6,93.34 78.6,93.03 78.28,92.71 77.33,92.71 | 77.33,92.71 74.59,92.71 R12.2 | T12.2 77.28,92.67 77.33,92.71 | R12.2 72.44,92.84 70.34,94.93 69.2,94.93 v69.14,95 64.25,95 62.72,96.52 62.72,98.51 U1.GND | 125.02,92.53 125.4,92.53 | 125.4,92.53 125.4,92.58 | 125.4,92.58 125.4,95.96 124.66,96.7 124.66,98.42 125.57,99.34 127.28,99.34 128.22,98.4 128.22,96.72 127.38,95.88 127.38,91.62 127.4,91.59 | 125.37,91.59 125.37,92.56 125.4,92.58 | 125.4,92.53 125.4,91.59
  Top 0.61: C2.1 C1.1 131.81,101.41 v131.62,101.6
  Top 0.813: C11.P$1 15.54,73.66 14.53,72.64 13.51,72.64 | R28.1 10.59,73.28 11.22,72.64 11.48,72.64 | 11.48,72.64 13.51,72.64 | 32.81,75.69 v32.56,75.44 | 11.48,72.64 11.22,72.39 11.22,67.12 C10.P$2 | 16.37,56.71 14.78,56.71 14.27,56.2 v14.27,54.61 | C4.1 36.94,75.25 U$2.OUT- U$2.IN- | v13.51,68.58 13.51,72.64 | R12.2
  Bottom 0.406: 96.81,57.39 v96.57,57.15 | 96.81,70.6 v97.01,70.8 | U$1.GND v94.79,95.57
  Bottom 0.61: v151.18,57.15 v132.89,57.15 v113.59,57.15 v96.57,57.15 v78.79,57.15 v61.01,57.15 60.06,56.2 v41.7,56.2 | 32.94,75.82 v32.56,75.44 | GND_2.1 71.93,97.79 v69.14,95 | GND_4.1 84.63,100.33 84.95,100.01 84.95,96.84 84.31,96.2 82.72,96.2 79.87,93.34 v78.6,93.34
  Bottom 0.813: 32.94,75.82 33.83,76.71 33.83,91.44 65.58,91.44 v69.14,95 | v26.72,56.9 41.45,56.9 41.45,56.45 v41.7,56.2 | v26.72,56.9 23.99,59.63 23.99,63.5 25.89,65.41 31.61,65.41 33.51,67.31 33.51,73.66 32.56,74.61 v32.56,75.44 | 14.27,56.83 14.27,57.91 11.22,60.96 11.22,66.29 v13.51,68.58 | 14.27,56.83 v14.27,54.61 10.97,54.61 4.62,48.26 v4.62,33.78 6.65,33.78 9.19,31.24 9.19,9.4 GND.1 | v26.72,56.9 14.34,56.9 14.27,56.83
  Bottom 0.93: v123.89,95.02 v123.89,100.1 | v123.89,100.1 v128.97,100.1 v128.97,95.02 | v118.67,101.35 122.64,101.35 v123.89,100.1
  other vias: 124.8,93.04 128,93.04 122.6,96.84 122.6,98.24 130.2,96.84 130.2,98.24 127,101.44 125.6,101.44 32.88,79.69 34.47,80.96 19.23,88.58 19.23,91.12 18.91,98.74 25.26,102.23 2.08,89.85 2.08,92.39 2.08,94.93 2.08,97.47 2.08,100.01 2.08,87.31 13.19,78.11 8.75,72.07 11.29,72.07 13.83,72.07 4.94,50.48 4.94,47.94 3.03,49.21 4.62,39.37 4.62,36.83 3.03,38.1 86.85,68.26 84.31,68.26 81.77,68.26 79.23,68.26 76.69,68.26 70.98,66.99 70.98,69.53 68.44,74.61 68.44,72.07 68.44,69.53 68.44,66.99 111.3,83.82 111.3,93.98 113.84,93.98 116.38,93.98 118.92,93.98 121.46,93.98 120.19,95.88 120.19,98.42 111.3,91.44 108.76,93.98 106.22,93.98 102.09,94.93 104.63,94.93 113.84,91.44 121.46,101.6 131.62,99.69 118.92,83.82 121.46,83.82 124,83.82 126.54,83.82 129.08,83.82 131.62,83.82 134.16,83.82 131.62,81.28 129.08,81.28 126.54,81.28 124,81.28 121.46,81.28 118.92,81.28 118.92,78.74 118.92,76.2 121.46,76.2 121.46,78.74 124,78.74 124,76.2 126.54,76.2 126.54,78.74 129.08,76.2 129.08,78.74 131.62,78.74 131.62,76.2 134.16,76.2 134.16,81.28 134.16,78.74 116.38,68.58 113.84,68.58 113.84,66.04 116.38,66.04 116.38,63.5 118.92,63.5 121.46,63.5 124,63.5 126.54,63.5 129.08,63.5 129.08,60.96 131.62,60.96 134.16,60.96 136.7,60.96 129.08,58.42 129.08,55.88 149.4,71.12 146.86,71.12 146.86,73.66 146.86,76.2 149.4,76.2 149.4,73.66 151.94,71.12 154.48,71.12 162.1,96.52 164.64,96.52 164.64,99.06 162.1,99.06 159.56,99.06 157.02,99.06 146.86,96.52 146.86,93.98 144.32,93.98 140.83,98.42 140.83,95.88 149.4,93.98 149.4,96.52 151.94,96.52 151.94,93.98 146.86,91.44 149.08,103.19 151.62,103.19 59.23,75.25 56.69,75.25 54.15,75.25 49.07,75.25 51.61,75.25 46.53,75.25 46.53,77.79 43.99,77.79 43.99,77.79 41.45,77.79 46.53,72.71 51.61,72.71 49.07,72.71 54.15,72.71 56.69,72.71 59.23,72.71 64.31,72.71 61.77,72.71 38.91,77.79 34.47,76.2 34.47,73.66 40.18,79.38 40.18,81.91 49.07,77.79 51.61,77.79 46.53,80.33 43.99,80.33 16.37,72.07 19.23,76.2 21.77,76.2 20.81,74.61 16.37,69.53 46.53,70.17 46.53,67.63 49.07,67.63 51.61,67.63 54.15,67.63 56.69,67.63 59.23,67.63 61.77,67.63 64.31,67.63 64.31,70.17 61.77,70.17 59.23,70.17 56.69,70.17 54.15,70.17 49.07,70.17 51.61,70.17 43.99,67.63 41.45,67.63 36.37,67.63 38.91,67.63 33.83,67.63 6.84,99.69 9.38,99.69 11.92,99.69 14.46,99.69 14.46,97.16 14.46,92.07 11.92,92.07 9.38,92.07 6.84,92.07 14.46,94.61 11.92,94.61 11.92,97.16 9.38,97.16 9.38,94.61 6.84,94.61 6.84,97.16 26.53,79.38 19.23,93.66 18.91,96.2 21.77,91.12 24.3,91.12 26.84,91.12 26.84,93.66 24.3,93.66 21.77,93.66 21.77,88.58 24.3,88.58 26.84,88.58 12.24,8.89 9.7,8.89 14.78,8.89 17.32,8.89 17.32,6.35 19.86,6.35 19.86,6.35 19.86,3.81 17.32,6.35 17.32,3.81 4.62,3.81 4.62,6.35 4.62,8.89 4.62,11.43 2.08,11.43 2.08,8.89 2.08,6.35 2.08,3.81 4.62,13.97 9.7,11.43 12.24,11.43 14.78,11.43 12.24,13.97 9.7,13.97 12.24,16.51 9.7,16.51 46.53,60.33 49.07,60.33 54.15,60.33 51.61,60.33 34.47,98.74 37.01,98.74 37.01,101.28 34.47,101.28 32.88,93.66 32.88,91.12 37.96,96.2 59.55,95.25 62.09,95.25 64.63,95.25 67.17,95.25 64.94,97.47 64.94,100.01 57.01,95.25 54.47,95.25
  pour Top: 0.05,105.16 169.2,105.16 169.2,0.04 0.05,0.04
  pour Bottom: 0,105.16 169,105.16 169,0.04 0,0.04
MCU_RX1  (via drill 0.5 pad 1.68, 0.6 pad 1.68)
  Top 0.406: 48.56,98.63 48.56,96.39 53.52,91.44 68.37,91.44 v68.69,91.12 70.03,91.12 72.25,88.9 v72.25,82.87 | IC3.9 87.31,78.88 86.53,78.11 83.04,78.11 v80.82,75.88
  Top 0.813: 48.56,98.63 U1.TXD0
  Bottom 0.406: v72.25,82.87 73.83,82.87 v80.82,75.88
  Bottom 0.61: MCU_RX1.1 74.47,96.52 69.07,91.12 v68.69,91.12
MCU_RX2  (via drill 0.5 pad 1.68)
  Top 0.406: v89.08,74.61 89.08,77.19 IC3.11
  Top 0.61: IC1.9 112.93,79.4 111.81,80.52 111.75,80.52 109.08,83.18 v105.9,83.18
  Top 0.813: v66.09,102.11 46.53,102.11 43.48,99.06 43.48,94.49 48.82,89.15 64.31,89.15 69.07,84.39 v69.07,83.18
  Bottom 0.61: v105.9,83.18 96.38,83.18 v89.08,74.61 87.81,74.61 85.9,72.71 70.03,72.71 69.71,73.02 69.71,76.83 69.07,77.47 v69.07,83.18
  Bottom 0.813: v66.09,102.11 68.88,102.11 MCU_RX2.1
MCU_TX1  (via drill 0.5 pad 1.68, 0.6 pad 1.68)
  Top 0.406: U1.RXD0 50.66,98.57 50.66,96.52 54.15,93.03 69.71,93.03 73.83,88.9 73.83,80.01 73.52,79.69 v72.88,79.69 | IC3.10 87.78,78.08 87.17,77.47 87.17,74.93 85.58,73.34 72.56,73.34 v71.61,74.3
  Bottom 0.61: v71.61,74.3 71.61,78.42 v72.88,79.69
MCU_TX2  (via drill 0.5 pad 1.68)
  Top 0.406: v89.39,72.39 90.79,73.79 IC3.12
  Top 0.61: IC1.10 112.48,78.4 111.55,77.47 111.55,74.87 v109.71,73.02
  Bottom 0.61: v109.71,73.02 90.03,73.02 v89.39,72.39
MISO  (via drill 0.5 pad 1.68)
  Top 0.406: IC3.2 87.46,84.48 86.22,85.72 86.22,90.49 91.61,95.88 91.61,98.74 87.81,102.55 87.81,102.87 v88.44,103.5
  Bottom 0.406: U$1.MISO 99.87,101.92 97.97,103.82 88.76,103.82 v88.44,103.5
MOSI  (via drill 0.5 pad 1.68)
  Top 0.406: IC3.1 87.61,85.28 86.85,86.04 86.85,90.17 92.57,95.88 92.57,96.52 93.52,97.47 96.06,97.47 96.69,96.84 v97.33,96.84
  Bottom 0.406: v97.33,96.84 U$1.MOSI
N$1
  Top 0.813: T1.1 18.27,58.1 18.84,58.67 R1.2
N$2  (via drill 0.5 pad 1.68)
  Top 0.813: v12.49,51.82 17.07,51.82 | 17.07,51.82 18.83,51.82 D1.A | T1.3 17.32,52.07 17.07,51.82
  Bottom 0.813: K1.2 11.82,39.03 9.7,41.15 9.7,49.02 v12.49,51.82
N$3
  Bottom 0.813: K1.S 23.76,38.77 26.97,35.56 26.97,17.97 33.83,11.11 K_1_NC.1
N$4
  Bottom 0.813: K1.P 17.79,19.53 28.75,8.57 K_1_IN.1
N$5
  Bottom 0.813: K1.O 13.78,44.18 14.78,43.18 14.78,13.97 K_1_C.1
N$6
  Top 0.813: T2.1 30.97,57.59 31.8,58.42 R2.2
N$7  (via drill 0.5 pad 1.68)
  Top 0.813: D2.A 31.27,51.56 v29.51,51.56 30.02,52.07 T2.3
  Bottom 0.813: K2.2 29.64,35.43 26.97,38.1 26.97,49.02 v29.51,51.56
N$8
  Bottom 0.813: K2.P 35.61,21.72 43.99,13.34 K_2_IN.1
N$9
  Bottom 0.813: K2.O 29.64,37.47 32.56,34.54 32.56,18.1 38.91,11.75 K_2_C.1
N$10
  Bottom 0.813: K2.S 41.58,37.02 44.31,34.29 44.31,27.94 49.07,23.18 K_2_NC.1
N$11
  Top 0.406: T3.1 51.65,56.98 R3.2
N$12  (via drill 0.5 pad 1.68)
  Top 0.61: T3.3 47.8,52.32 v47.29,51.82
  Top 0.813: v47.29,51.82 49.31,51.82 D3.A
  Bottom 0.813: K3.2 47.16,34.92 44.5,37.59 44.5,49.02 v47.29,51.82
N$13
  Bottom 0.813: K3.P 53.13,25.46 59.23,19.37 K_3_IN.1
N$14
  Bottom 0.813: K3.O 47.16,37.72 50.34,34.54 50.34,24.77 54.15,20.95 K_3_C.1
N$15
  Bottom 0.813: K3.S 59.1,37.21 62.28,34.04 62.28,25.15 64.31,23.11 K_3_NC.1
N$16
  Top 0.61: R4.2 67.97,58.42 T4.1
N$17  (via drill 0.5 pad 1.68)
  Top 0.61: T4.3 65.58,53.59 v64.06,52.07
  Top 0.813: v64.06,52.07 67.34,52.07 D4.A
  Bottom 0.813: K4.2 64.94,34.92 62.02,37.85 62.02,50.04 v64.06,52.07
N$18
  Bottom 0.813: K_4_IN.1 74.47,26.29 K4.P
N$19
  Bottom 0.813: K4.O 64.94,37.47 66.85,35.56 66.85,26.42 69.39,23.88 K_4_C.1
N$20
  Bottom 0.813: K4.S 76.88,39.5 79.55,36.83 K_4_NC.1
N$21
  Top 0.61: R5.2 85.75,58.42 T5.1
N$22  (via drill 0.5 pad 1.68)
  Top 0.61: T5.3 83.36,52.07 v83.11,51.82
  Top 0.813: v83.11,51.82 84.87,51.82 D5.A
  Bottom 0.813: K5.2 82.72,37.72 79.8,40.64 79.8,48.51 v83.11,51.82
N$23
  Bottom 0.813: K_5_IN.1 89.71,28.83 K5.P
N$24
  Bottom 0.813: K5.O 82.72,41.53 85.9,38.35 85.9,25.15 84.63,23.88 K_5_C.1
N$25
  Bottom 0.813: K5.S 94.66,43.56 91.49,40.39 91.49,16 94.79,12.7 K_5_NC.1
N$26
  Top 0.61: R6.2 103.53,58.42 T6.1
N$27  (via drill 0.5 pad 1.68)
  Top 0.61: T6.3 101.14,52.32 v101.9,51.56
  Top 0.813: D6.A 103.68,53.34 v101.9,51.56
  Bottom 0.813: v101.9,51.56 101.9,48.77 104.19,46.48 104.19,35.31 K6.2
N$28
  Bottom 0.813: K_6_IN.1 104.95,28.07 K6.P
N$29
  Bottom 0.813: K6.O 100.76,41.27 98.09,38.61 98.09,26.92 99.87,25.15 K_6_C.1
N$30
  Bottom 0.813: K_6_NC.1 110.03,35.05 113.08,38.1 113.08,43.69 K6.S
N$31
  Top 0.61: T7.1 120.02,56.98 121.46,58.42 R7.2
N$32  (via drill 0.5 pad 1.68)
  Top 0.61: T7.3 v118.92,51.56
  Top 0.813: v118.92,51.56 120.17,51.56 D7.A
  Bottom 0.813: K7.2 120.95,34.29 120.95,49.53 v118.92,51.56
N$33
  Bottom 0.813: K_7_IN.1 120.19,25.53 K7.P
N$34
  Bottom 0.813: K7.O 118.54,37.47 115.87,34.8 115.87,5.84 K_7_C.1
N$35
  Bottom 0.813: K7.S 130.48,38.99 127.81,36.32 127.81,14.92 125.27,12.38 K_7_NC.1
N$36
  Top 0.61: R8.2 140.11,58.42 T8.1
N$37  (via drill 0.5 pad 1.68)
  Top 0.61: T8.3 137.72,51.56 v137.46,51.31
  Top 0.813: v137.46,51.31 138.97,51.31 D8.A
  Bottom 0.813: K8.2 139.24,34.8 139.24,49.53 v137.46,51.31
N$38
  Bottom 0.813: K8.P 142.29,29.4 137.65,24.77 137.65,12.7 135.75,10.79 135.75,5.4 K_8_IN.1
N$39
  Bottom 0.813: K8.O 136.32,37.21 133.65,34.54 133.65,14.73 130.35,11.43 K_8_C.1
N$40
  Bottom 0.813: K8.S 148.26,38.73 145.08,35.56 145.08,28.45 142.8,26.16 142.8,14.35 140.51,12.07 K_8_NC.1
N$41
  Top 0.61: R9.2 156.87,58.42 T9.1
N$42  (via drill 0.5 pad 1.68)
  Top 0.61: T9.3 v154.48,51.56
  Top 0.813: v154.48,51.56 155.73,51.56 D9.A
  Bottom 0.813: K9.2 154.1,37.21 157.02,40.13 157.02,49.02 v154.48,51.56
N$43
  Bottom 0.813: K_9_IN.1 150.67,20.45 K9.P
N$44
  Bottom 0.813: K9.O 151.43,41.4 151.43,26.42 145.59,20.57 K_9_C.1
N$45
  Bottom 0.813: K9.S 163.37,41.4 163.37,27.43 156.64,20.7 156.26,20.32 155.75,19.81 K_9_NC.1
N$46  (via drill 0.5 pad 1.68)
  Top 0.61: v27.16,61.59 R10.2 19.04,60.77 17.32,59.05 10.34,59.05 9.7,58.42 C5.2
  Top 0.813: U$2.IN+ 66.22,60.64 v68.12,62.55
  Bottom 0.813: v68.12,62.55 29.38,62.55 28.43,61.59 v27.16,61.59
N$47
  Top 0.61: U$2.OUT+ 37.78,60.64 D12.A
N$48
  Top 0.61: R10.1 5.57,61.59 3.35,59.37 IC2.1
N$49  (via drill 0.5 pad 1.68)
  Top 0.406: IC3.42 92.39,89.08 91.93,89.53 v89.39,89.53
  Bottom 0.61: v89.39,89.53 78.28,89.53 77.01,90.8 77.01,99.06 SDO.1
N$50  (via drill 0.5 pad 1.68)
  Top 0.406: R11.2 79.69,95.94 v79.55,96.07 74.91,96.07 R12.1
  Bottom 0.61: 3V3.1 82.09,101.28 79.55,98.74 v79.55,96.07
N$51
  Top 0.406: R13.2 103.71,92.71 T10.1
N$52
  Top 0.406: IC1.1 115.08,87.31 110.64,87.31 T10.3
N$53
  Top 0.61: IC5.2 8.91,84.95 D15.K
  Top 0.813: 10.18,84.25 D15.K | IC5.2 8.91,89.06 8.43,89.53 4.62,89.53 3.99,90.17 3.99,100.96 5.26,102.23 22.08,102.23 23.42,100.9 L1.P$1
N$54
  Bottom 1.016: D10.A 7.16,6.35 12V.1
N$55
  Top 0.406: R14.1 66.53,80.01 66.53,79.06 67.48,78.11 73.83,78.11 74.47,78.74 74.47,88.58 75.08,89.2 T12.3
  Top 0.61: U1.RESET 48.58,84.35 49.32,85.09 52.12,85.09 52.63,84.58 52.63,82.3 U1.CH_PD 52.56,82.23 52.56,80.01 53.52,79.06 64.94,79.06 66.03,80.14 R14.1
N$56  (via drill 0.5 pad 1.68)
  Top 0.813: U$2.B+ 34.15,64.45 v30.66,67.94
  Bottom 0.813: v30.66,67.94 28.75,69.85 4V8.1
N$57
  Top 0.406: R15.2 74.15,66.33 74.15,70.8 74.79,71.44 75.91,71.44 T11.1
N$58  (via drill 0.5 pad 1.68)
  Top 0.813: U$2.B- v31.61,71.44
  Bottom 0.813: v31.61,71.44 30.66,72.39 30.66,98.74 31.29,99.38 GND_3.1
N$59  (via drill 1.6 pad 2.54)
  other vias: 2.99,103.19
N$60
  Top 0.61: 21.13,81.15 R26.2
  Top 0.813: C12.2 6.53,74.51 6.53,66.04 8.11,64.45 14.78,64.45 16.37,66.04 D11.A 17.64,66.21 17.64,67.63 23.67,73.66 C11.P$2 25.26,73.85 25.26,76.83 21.07,81.03 R26.2 23.42,83.44 L1.P$2 23.35,85.09 19.23,85.09 17.7,83.57 R27.2
N$61  (via drill 0.6 pad 1.68)
  Top 0.406: C15.1 v80.82,83.18 80.82,82.23 83.04,80.01 85.58,80.01 86.05,80.48 IC3.7
  Bottom 0.406: v80.82,83.18 82.41,83.18 Q1.2
N$62
  Top 0.406: T12.1 77.28,86.38 R20.2
N$63
  Top 0.61: R26.1 17.95,80.77 R27.1 15.09,80.96 13.83,80.96 13.19,81.6 13.19,84.77 12.24,85.72 12.24,87.26 IC5.4
  Top 0.813: R28.2 15.03,74.93 18.34,78.23 18.34,80.9 R26.1
N$64
  Top 0.8: IC1.60 126.41,92.36 126.4,92.37
  Top 0.93: 126.4,92.37 126.4,97.54 ANT.1
N$65
  Top 0.61: IC1.52 138.76,90.65 141.46,87.95 141.46,85.66 R21.1
N$66
  Top 0.61: R21.2 147.05,85.6 153.84,92.39 153.84,99.78 T13.1
N$67  (via drill 0.5 pad 1.68)
  Top 0.61: T13.3 149.97,100.77 v149.65,100.46
  Bottom 0.61: LED_GND.1 148.51,101.6 v149.65,100.46
N$68  (via drill 0.5 pad 1.68)
  Top 0.61: R22.1 141.78,101.41 v142.1,101.09
  Bottom 0.61: v142.1,101.09 143.81,101.09 LED_3V.1
N$69
  Top 0.406: IC1.30 130.41,65.72 130.73,65.41 131.11,65.02 132.89,63.25 160.83,63.25 162.23,64.64 | 162.23,64.64 162.35,64.77 162.35,68.53 X2.C1 | C9.2 164.89,61.98 162.23,64.64
N$70
  Top 0.406: X2.C2 159.66,65.3 R23.2
N$71
  Top 0.406: R24.2 156.26,67.82 X2.C3
N$72
  Top 0.61: X2.C7 157.02,94.28 157.02,92.07 147.96,83.02 147.96,80.8 146.54,79.38 144.11,79.38 C8.2 R25.1
N$73
  Top 0.406: IC1.33 133.41,66.28 134.41,65.28 R23.1
N$74
  Top 0.406: IC1.32 132.41,70.13 132.64,70.36 135.18,70.36 137.72,67.82 R24.1
N$75
  Top 0.406: IC1.31 131.41,70.66 131.87,71.12 135.43,71.12 136.19,70.36 142.61,70.36 144,71.75 144,73.53 R25.2
N$76  (via drill 1.6 pad 2.54)
  other vias: 165,103.19
N$77  (via drill 1.6 pad 2.54)
  other vias: 165,19.24
N$78  (via drill 1.6 pad 2.54)
  other vias: 3,19.24
N$79  (via drill 0.6 pad 1.68)
  Top 0.406: IC3.8 86.84,79.68 86.22,79.06 81.14,79.06 v80.82,79.38 79.55,80.64 C16.1
  Bottom 0.406: Q1.1 84.31,76.52 81.45,79.38 v80.82,79.38
N$80
  Top 0.406: IC3.34 98.79,88.14 98.92,88.27 ADC.1
PWRKEY
  Top 0.406: IC3.40 93.99,92.29 R13.1
RELAY_1  (via drill 0.5 pad 1.68)
  Top 0.406: IC3.14 92.39,71.89 90.03,69.53 v90.03,66.67
  Top 0.813: R1.1 29,58.67 v30.34,60.01
  Bottom 0.406: v30.34,60.01 30.02,59.69 26.21,59.69 25.57,60.33 25.57,62.87 26.84,64.14 33.2,64.14 34.47,65.41 88.76,65.41 v90.03,66.67
RELAY_2  (via drill 0.5 pad 1.68)
  Top 0.406: R2.1 55.42,58.42 61.45,64.45 70.03,64.45 v70.66,63.82 | v92.57,66.67 92.57,71.12 93.19,71.74 | 93.19,71.74 93.2,71.75 | IC3.15 93.19,71.74
  Bottom 0.406: v70.66,63.82 90.98,63.82 92.57,65.41 v92.57,66.67
RELAY_3  (via drill 0.5 pad 1.68)
  Top 0.406: R3.1 54.6,57.28 58.09,57.28 59.55,58.74 66.53,58.74 68.75,60.96 v70.98,60.96 | v94.79,68.58 94.79,71.44 93.99,72.24 IC3.16
  Bottom 0.406: v94.79,68.58 94.79,65.41 90.34,60.96 v70.98,60.96
RELAY_4  (via drill 0.5 pad 1.68)
  Top 0.406: R4.1 v74.47,58.42 | IC3.21 97.99,72.73 97.97,72.71 99.23,71.44 99.23,68.9 97.65,67.31 v97.65,65.72
  Bottom 0.406: v74.47,58.42 91.93,58.42 97.65,64.14 v97.65,65.72
RELAY_5  (via drill 0.5 pad 1.68)
  Top 0.406: R5.1 91.93,58.42 93.52,60.01 106.22,60.01 v107.49,61.28 | v101.78,68.58 101.78,69.85 98.79,72.83 IC3.22
  Bottom 0.406: v101.78,68.58 107.49,62.87 v107.49,61.28
RELAY_6
  Top 0.406: R6.1 108.76,58.42 110.35,60.01 110.35,68.58 101.65,77.28 IC3.23
RELAY_7
  Top 0.406: R7.1 125.4,59.56 124,60.96 115.43,60.96 111.3,65.09 111.3,68.9 102.12,78.08 IC3.24
RELAY_8  (via drill 0.5 pad 1.68)
  Top 0.406: v105.58,77.47 104.17,78.88 IC3.25
  Top 0.61: R8.1 144.32,58.54 145.97,58.54 v146.86,59.44
  Bottom 0.61: v146.86,59.44 146.86,61.21 137.18,70.89 137.18,70.95 136.06,72.07 112.89,72.07 107.49,77.47 v105.58,77.47
RELAY_9  (via drill 0.5 pad 1.68)
  Top 0.406: v107.49,79.38 107.17,79.69 100.6,79.69 IC3.26
  Top 0.61: R9.1 160.83,58.55 160.83,60.2 160.32,60.71 v150.16,60.71
  Bottom 0.61: v150.16,60.71 150.16,63.25 139.98,73.43 113.44,73.43 v107.49,79.38
RESET  (via drill 0.5 pad 1.68)
  Top 0.406: IC3.4 87.16,82.88 84.63,85.41 84.63,90.17 84.31,90.49 82.93,90.49 R17.2 82.88,92.88 v82.72,93.03
  Bottom 0.406: U$1.RST 94.47,101.6 91.61,98.74 91.61,95.57 90.34,94.3 83.36,94.3 82.72,93.66 v82.72,93.03
SCK  (via drill 0.5 pad 1.68)
  Top 0.406: v89.08,96.84 89.08,94.3 85.58,90.8 85.58,85.41 87.31,83.68 IC3.3
  Bottom 0.406: U$1.SCK 95.74,103.19 92.89,103.19 89.08,99.38 v89.08,96.84
VCC_DETECT
  Top 0.406: IC3.13 91.59,72.05 88.76,69.22 81.14,69.22 80.61,69.74 R16.2 80.61,71.12 79.89,70.41 T11.3

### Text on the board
Top: jTech | HCM-R9-I0 | jTech - Home Control Module
Bottom: BOTTOM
